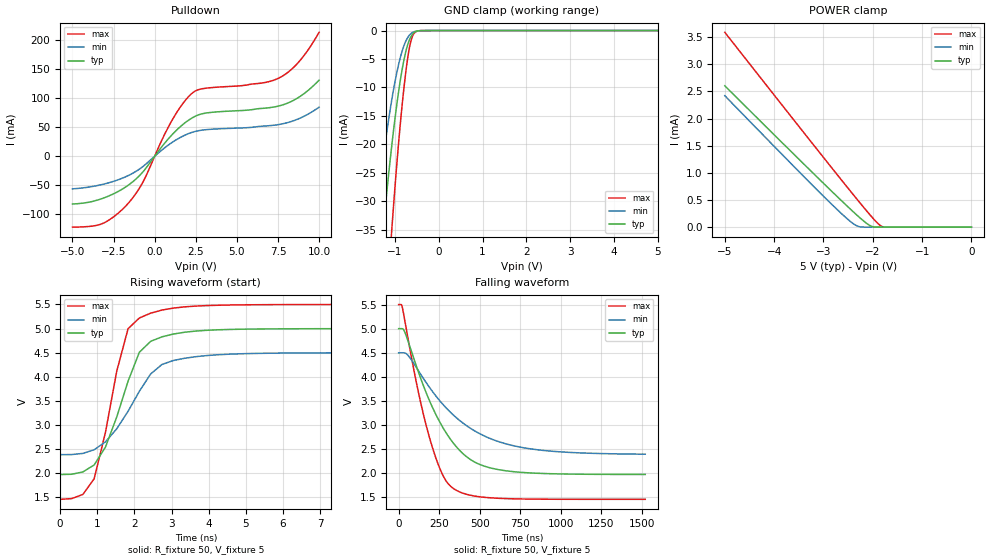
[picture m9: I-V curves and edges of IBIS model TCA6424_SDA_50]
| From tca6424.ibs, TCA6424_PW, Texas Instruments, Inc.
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[Model]   TCA6424_SDA_50
Model_type  I/O_open_drain
Vinl=1.35
Vinh=3.85
Enable   Active-Low
Vref =   0
Rref =   500
Cref =   50p
Vmeas =   2.5
| variable   typ   min   max
C_comp   3.07pF   2.25pF   3.43pF
| C_pulldown   1.95pF   0.73pF   2.54pF
| C_tri-state   3.07pF   2.25pF   3.43pF
[Temperature Range]   40   100   -40
| Ambient temperature   25   85   -40
[Voltage range]   5   4.5   5.5
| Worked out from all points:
|   slope of the pulldown table from 0 to 0.75 V, typ, clamps not added: 27.4 ohm
|   GND clamp passes 1 mA (typ) near -0.63 V on its own axis
|   POWER clamp passes 1 mA (typ) near -3.22 V on its own axis
|   rising waveform, R_fixture 50, V_fixture 5: 20-80 % time 837ps typ, 1.07ns min, 686ps max; typ from 1.98 V to 5 V
|   falling waveform, R_fixture 50, V_fixture 5: 20-80 % time 256ns typ, 371ns min, 171ns max; typ from 5 V to 1.98 V
[GND Clamp]
| TCA6424_SDA_50
|   Voltage   I(typ)   I(min)   I(max)
-5V       -485.8mA   -373.6mA   -646.6mA
-1.49V    -54.18mA   -36.17mA   -85.83mA
-1.445V   -50.02mA   -33.15mA   -79.8mA
-1.275V   -35.24mA   -22.59mA   -58.03mA
-1.085V   -20.86mA   -12.62mA   -36.07mA
-1.065V   -19.51mA   -11.7mA    -33.94mA
-930mV    -11.31mA   -6.333mA   -20.71mA
-795mV    -5.103mA   -2.618mA   -9.933mA
-680mV    -1.802mA   -894.8uA   -3.358mA
-585mV    -504.4uA   -278.7uA   -738.2uA
-405mV    -14.47uA   -12.15uA   -11.55uA
5V        759.7pA    2.316nA    213.9pA
[POWER Clamp]
| TCA6424_SDA_50
|   Voltage   I(typ)   I(min)   I(max)
-5V       2.602mA    2.42mA     3.587mA
-3.24V    1.021mA    787.9uA    1.559mA
-2.49V    362.7uA    132.2uA    704.6uA
-2.3V     203.7uA    16.21uA    492uA
-2.08V    42.03uA    34.52nA    251.7uA
-1.99V    6.377uA    6.606nA    157.9uA
-1.86V    68.52nA    4.495nA    39.19uA
-1.805V   10.53nA    4.332nA    9.164uA
-1.735V   2.411nA    4.161nA    409.2nA
0V        0A         0A         0A
[Pulldown]
| TCA6424_SDA_50
|   Voltage   I(typ)   I(min)   I(max)
-5V       -82.53mA   -56.3mA    -122.4mA
-3.17V    -72.74mA   -48.6mA    -116.1mA
-1.63V    -50.43mA   -33.63mA   -81.91mA
-695mV    -26.31mA   -17.3mA    -43.63mA
465mV     17.55mA    11.31mA    29.55mA
1.13V     39.3mA     25.14mA    65.7mA
2.315V    66.7mA     41.58mA    109.6mA
3.235V    75mA       46.11mA    117.8mA
6.5V      82.47mA    51.75mA    126.3mA
7.53V     86.58mA    54.63mA    134.6mA
8.745V    101.4mA    64.52mA    162.1mA
10V       131.3mA    84.61mA    213.8mA
[Ramp]
| TCA6424_SDA_50
| variable   typ   min   max
dV/dt_r   1.82/8.21E-10   1.27/1.05E-09   2.42/6.28E-10
dV/dt_f   1.82/2.56E-07   1.26/3.71E-07   2.42/1.71E-07
R_load = 50
[Rising Waveform]
| TCA6424_SDA_50
R_fixture =   50
C_fixture =   0
L_fixture =   0
V_fixture =   5
V_fixture_min = 4.5
V_fixture_max = 5.5
|   Time   V(typ)   V(min)   V(max)
0s        1.976V     2.389V     1.461V
613ps     2.028V     2.412V     1.562V
917ps     2.173V     2.489V     1.888V
1.221ns   2.545V     2.652V     2.851V
1.525ns   3.169V     2.923V     4.12V
1.829ns   3.909V     3.286V     4.998V
2.133ns   4.509V     3.7V       5.22V
3.045ns   4.887V     4.338V     5.425V
5.781ns   4.995V     4.491V     5.497V
1.52us    5V         4.5V       5.5V
[Falling Waveform]
| TCA6424_SDA_50
R_fixture =   50
C_fixture =   0
L_fixture =   0
V_fixture =   5
V_fixture_min = 4.5
V_fixture_max = 5.5
|   Time   V(typ)   V(min)   V(max)
0s        5V         4.5V       5.5V
22.2ns    5V         4.501V     5.45V
118ns     4.14V      4.149V     3.743V
196.7ns   3.456V     3.752V     2.665V
267.2ns   2.981V     3.452V     1.998V
329.2ns   2.661V     3.234V     1.706V
455.7ns   2.259V     2.906V     1.536V
623.5ns   2.072V     2.65V      1.481V
941.8ns   1.992V     2.459V     1.463V
1.52us    1.977V     2.397V     1.461V
